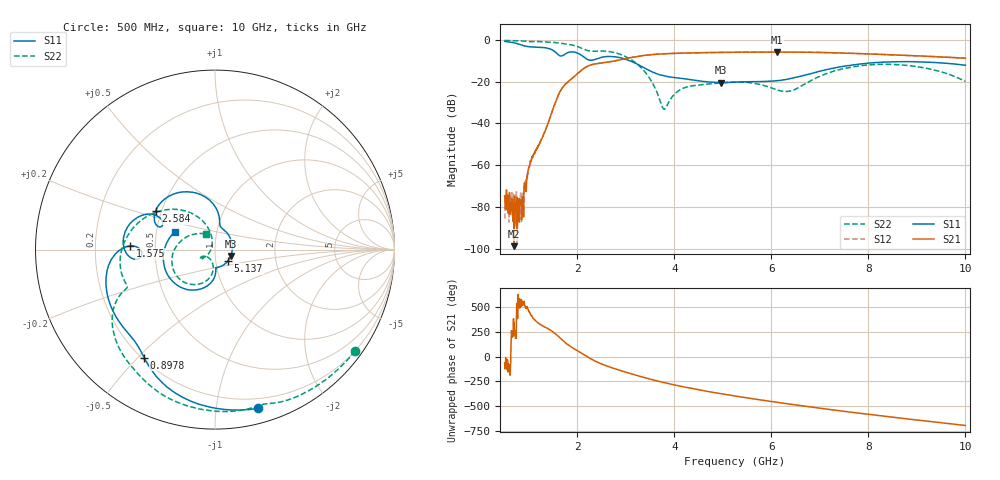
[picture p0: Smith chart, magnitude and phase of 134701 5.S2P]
!  2-Port S-parameters saved by WinCal
! VAR MeasName=S-Parameters (CALIBRATED_DATA) read from VNA (N5242A)
! VAR MeasDate=2013-7-3 16:21:49
! VAR NAME=134701 5
! VAR FILENAME=134701 5.S2P
! VAR DATE=2013-7-3 16:21:49
! VAR PHYS_PORTS=1,2
# Hz S MA R 50
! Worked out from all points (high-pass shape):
!   1601 points, 500 MHz to 10 GHz, reference 50 ohm
!   highest |S21| = -5.88 dB at 6.123 GHz (marker M1); lowest = -98.9 dB at 695.9 MHz (marker M2)
!   |S21| within 3 dB of the highest: 3.026 GHz to end of sweep
!   lowest |S11| = -20.5 dB at 4.965 GHz (marker M3), VSWR 1.21, Z = 59.4 - j4.33 ohm
!   |S11| at or under -10 dB: 3.077 GHz to end of sweep
!   |S22| runs from -33.3 to -0.3 dB; largest |S21 - S12| = 0.002
!   S11 on the Smith chart (normalised r, x): 500 MHz: 0.12, -1.30; 897.8 MHz: 0.21, -0.52; 1.575 GHz: 0.36, +0.02; 2.584 GHz: 0.46, +0.24; 5.137 GHz: 1.15, -0.14; 10 GHz: 0.62, +0.13
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5e8  0.9173 -74.8  0.0001821 -63.3  5.64e-05 -32.4  0.9631 -35.9
6.959375e8  0.8456 -101.5  1.139e-05 -19.3  0.0001408 -158.2  0.9519 -49.8
8.20625e8  0.7688 -116.3  0.0001253 -159.4  0.0001432 148.0  0.94 -58.8
8.978125e8  0.7195 -123.3  0.0002453 -162.6  0.0001581 -169.1  0.93 -64.3
1.040312e9  0.6749 -133.2  0.001286 64.2  0.001277 64.2  0.9023 -73.4
1.366875e9  0.6356 -162.9  0.008187 -71.2  0.008204 -71.5  0.8896 -96.7
1.574688e9  0.4743 177.5  0.0382 -140.9  0.03808 -141.1  0.8498 -112.8
2.085312e9  0.4249 152.3  0.1874 34.3  0.1866 34.2  0.63 -151.7
2.287188e9  0.3225 155.6  0.2521 -24.8  0.2511 -24.9  0.5325 -156.8
2.584062e9  0.395 146.8  0.2866 -90.9  0.2856 -90.8  0.5334 -172.6
3.237188e9  0.2598 93.1  0.3998 168.3  0.3996 168.4  0.2593 125.6
3.670625e9  0.1488 79.6  0.4541 111.3  0.4531 111.3  0.0446 110.4
3.795312e9  0.1359 77.9  0.4624 96.6  0.4621 96.7  0.02174 166.4
4.169375e9  0.1179 60.8  0.4791 56.6  0.4785 56.7  0.06832 -143.6
4.965e9  0.09456 -22.4  0.4985 -15.0  0.4994 -14.9  0.09269 -143.9
5.137188e9  0.0955 -40.7  0.5011 -28.9  0.5016 -28.9  0.09613 -144.7
5.25e9  0.09656 -50.9  0.5026 -37.8  0.5029 -37.8  0.09725 -145.8
6.122812e9  0.1049 -87.2  0.5083 -101.8  0.5082 -101.7  0.06287 -142.1
6.835312e9  0.1571 -91.7  0.5009 -150.2  0.5015 -150.2  0.1083 -95.1
7.53e9  0.2362 -110.8  0.4788 165.3  0.4793 165.3  0.2086 -113.8
8.420625e9  0.2949 -142.7  0.439 112.3  0.4378 112.2  0.2587 -152.5
1e10  0.2454 156.4  0.3631 24.8  0.3626 24.7  0.1008 120.0
